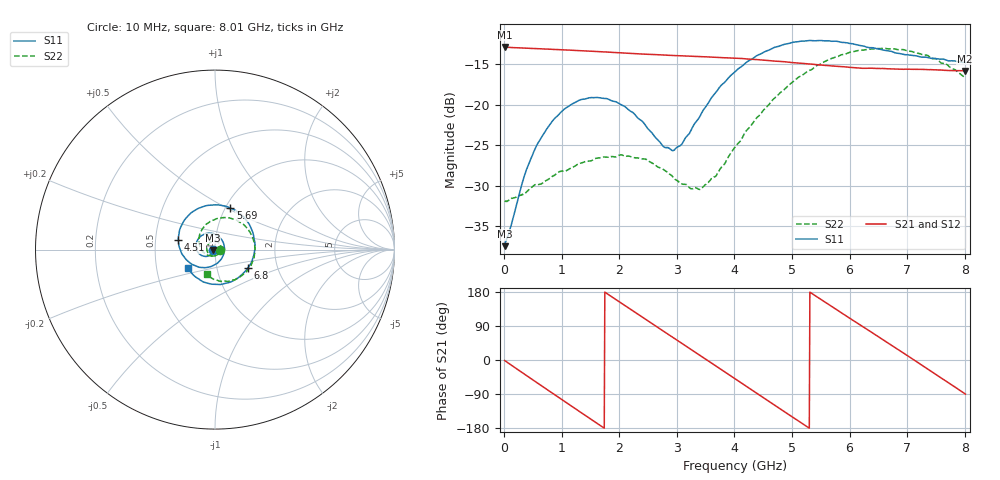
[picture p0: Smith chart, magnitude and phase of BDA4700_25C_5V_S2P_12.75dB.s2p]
!Agilent Technologies,E5071B,MY42404982,A.09.10
!Date: Mon Oct 20 13:32:31 2025
!Data & Calibration Information:
!Freq	S11:SOLT2(ON)	S21:SOLT2(ON)	S12:SOLT2(ON)	S22:SOLT2(ON)
# Hz S RI R 50
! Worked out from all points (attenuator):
!   801 points, 10 MHz to 8.01 GHz, reference 50 ohm
!   highest |S21| = -12.86 dB at 10 MHz (marker M1); lowest = -15.8 dB at 8 GHz (marker M2)
!   lowest |S11| = -37.5 dB at 10 MHz (marker M3), VSWR 1.03, Z = 48.7 - j0.155 ohm
!   |S11| at or under -10 dB: start of sweep to end of sweep
!   |S22| runs from -32.0 to -13.0 dB; largest |S21 - S12| = 0.0018
!   S11 on the Smith chart (normalised r, x): 10 MHz: 0.97, -0.00; 4.51 GHz: 0.66, +0.08; 5.69 GHz: 1.05, +0.52; 6.8 GHz: 1.41, -0.30; 8.01 GHz: 0.72, -0.15
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1e7  -0.0132 -0.00159  0.2275 -0.005  0.2276 -0.00515  0.0253 -0.000932
3.6e8  -0.0251 -0.0272  0.1768 -0.1376  0.1767 -0.1377  0.0214 -0.0184
5.8e8  -0.0432 -0.0373  0.1087 -0.1938  0.1088 -0.194  0.0133 -0.0293
8.8e8  -0.0755 -0.0327  -0.00641 -0.2197  -0.00649 -0.2197  -0.00924 -0.0355
1.35e9  -0.1063 0.0182  -0.1653 -0.1387  -0.1654 -0.1387  -0.0411 -0.0146
1.94e9  -0.0563 0.0878  -0.1972 0.073  -0.1973 0.0731  -0.0323 0.0349
2.33e9  0.00677 0.082  -0.1037 0.1786  -0.1037 0.1787  -0.000767 0.0468
2.68e9  0.0468 0.0375  0.0183 0.203  0.0183 0.2029  0.0255 0.0321
2.96e9  0.0504 -0.015  0.1107 0.1682  0.1108 0.1681  0.0332 0.0108
3.4e9  -0.00285 -0.0845  0.194 0.0423  0.1942 0.0422  0.0169 -0.0247
3.69e9  -0.0678 -0.0998  0.1878 -0.0573  0.1878 -0.0578  -0.0102 -0.0352
4.01e9  -0.1431 -0.0711  0.1262 -0.1475  0.1263 -0.1474  -0.0464 -0.0286
4.51e9  -0.2041 0.0549  -0.0337 -0.1857  -0.0337 -0.1859  -0.0879 0.031
4.96e9  -0.1512 0.1864  -0.1513 -0.103  -0.1513 -0.1036  -0.0724 0.1122
5.35e9  -0.0349 0.2468  -0.1774 0.0155  -0.1775 0.0149  -0.00508 0.1657
5.69e9  0.0851 0.2318  -0.1354 0.1088  -0.1354 0.1091  0.0792 0.1766
6.21e9  0.2096 0.0989  -0.00017 0.1681  0.00128 0.1685  0.1938 0.0987
6.68e9  0.2049 -0.0661  0.1211 0.1147  0.1213 0.1147  0.2198 -0.0278
6.8e9  0.1822 -0.1025  0.1415 0.0871  0.1421 0.0866  0.2126 -0.0596
7.36e9  0.0204 -0.1944  0.1503 -0.0679  0.1505 -0.068  0.1113 -0.168
8e9  -0.1512 -0.1026  0.0032 -0.162  0.00317 -0.1624  -0.0446 -0.1403
8.01e9  -0.153 -0.1001  0.000246 -0.162  0.000443 -0.1623  -0.0466 -0.1384
